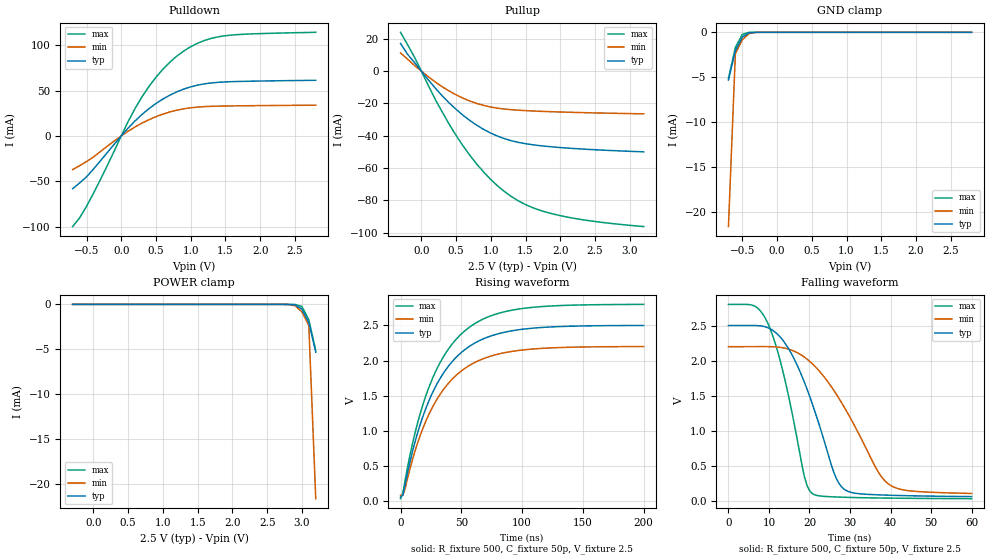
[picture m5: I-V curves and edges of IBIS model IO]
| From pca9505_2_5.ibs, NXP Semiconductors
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[Model]   IO
Model_type I/O
Vinh=1.5
Vinl=0.75
Vref=2.5
Vmeas=1.25
Rref=500
Cref=50p
C_comp   7p   6.8p   7.2p
[Temperature Range] 27   85   -40
[Voltage Range]   2.5   2.2   2.8
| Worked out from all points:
|   slope of the pulldown table from 0 to 0.375 V, typ, clamps not added: 13.2 ohm
|   slope of the pullup table from 0 to 0.375 V, typ, clamps not added: 20.2 ohm
|   GND clamp passes 1 mA (typ) near -0.53 V on its own axis
|   falling waveform, R_fixture 500, C_fixture 50p, V_fixture 2.5: 20-80 % time 8.89ns typ, 12.5ns min, 6.36ns max; typ from 2.5 V to 0.069 V
|   rising waveform, R_fixture 500, C_fixture 50p, V_fixture 2.5: 20-80 % time 36.2ns typ, 36.4ns min, 36ns max; typ from 0.055 V to 2.5 V
[Pullup]
-300mV    17.1mA     11.24mA    23.99mA
-100mV    5.385mA    3.536mA    8.641mA
100mV     -5.421mA   -3.476mA   -8.883mA
300mV     -15.3mA    -9.683mA   -25.27mA
500mV     -23.69mA   -14.69mA   -39.81mA
800mV     -33.57mA   -20.05mA   -57.68mA
1V        -38.39mA   -22.25mA   -67.13mA
1.2V      -41.86mA   -23.52mA   -74.66mA
1.5V      -44.93mA   -24.47mA   -82.61mA
1.9V      -46.95mA   -25.18mA   -88.44mA
2.4V      -48.44mA   -25.77mA   -92.46mA
3.2V      -49.96mA   -26.44mA   -96.19mA
[Pulldown]
-700mV    -58.3mA    -37.22mA   -100mA
-600mV    -51.97mA   -32.92mA   -90.55mA
-500mV    -45.2mA    -28.3mA    -77.83mA
-300mV    -27.54mA   -17.33mA   -48.27mA
100mV     8.694mA    5.192mA    15.93mA
300mV     23.71mA    14.14mA    43.15mA
500mV     35.71mA    21.18mA    64.7mA
800mV     48.56mA    28.33mA    87.97mA
1.1V      55.98mA    31.79mA    102.2mA
1.4V      59.1mA     32.83mA    109.3mA
1.8V      60.23mA    33.26mA    112.2mA
2.8V      61.29mA    33.85mA    114.3mA
[GND Clamp]
-700mV    -5.302mA   -21.58mA   -5.122mA
-600mV    -2.04mA    -2.358mA   -1.687mA
-500mV    -525.2uA   -816.9uA   -228.9uA
-400mV    -48.21uA   -135uA     -7.763uA
-200mV    -27.28nA   -200nA     -811.9pA
2.8V      51pA       210.6pA    36.58pA
[POWER Clamp]
-300mV    51pA       210.6pA    36.58pA
2.7V      -27.28nA   -200nA     -811.9pA
2.9V      -48.21uA   -135uA     -7.763uA
3V        -525.2uA   -816.9uA   -228.9uA
3.1V      -2.04mA    -2.358mA   -1.687mA
3.2V      -5.302mA   -21.58mA   -5.122mA
[Falling Waveform]
R_fixture=500
C_fixture=50p
V_fixture=2.5
V_fixture_min=2.2
V_fixture_max=2.8
0s        2.5V       2.2V       2.8V
6.667ns   2.5V       2.2V       2.77V
9.697ns   2.469V     2.2V       2.535V
15.15ns   2.14V      2.159V     1.412V
18.79ns   1.687V     2.049V     342.6mV
20.61ns   1.401V     1.962V     115.7mV
26.06ns   405mV      1.574V     64.59mV
29.09ns   154mV      1.288V     58.45mV
40ns      87.71mV    228.2mV    46.9mV
60ns      68.75mV    113.2mV    39.29mV
[Rising Waveform]
R_fixture=500
C_fixture=50p
V_fixture=2.5
V_fixture_min=2.2
V_fixture_max=2.8
0s        55.42mV    81.35mV    33.81mV
2.02ns    86.5mV     85.54mV    122.5mV
8.081ns   579.6mV    478.1mV    677.9mV
14.14ns   975.7mV    831.2mV    1.119V
24.24ns   1.462V     1.266V     1.659V
38.38ns   1.896V     1.655V     2.137V
54.55ns   2.176V     1.907V     2.446V
72.73ns   2.34V      2.054V     2.626V
98.99ns   2.442V     2.147V     2.737V
200ns     2.499V     2.199V     2.799V
[Ramp]
R_load=500
dV/dt_r   7.201E-3/2.268E-9   6.234E-3/2.629E-9   8.154E-3/1.897E-9
dV/dt_f   1.459E+0/5.747E-9   1.254E+0/8.481E-9   1.657E+0/4.049E-9
|[End   IO
